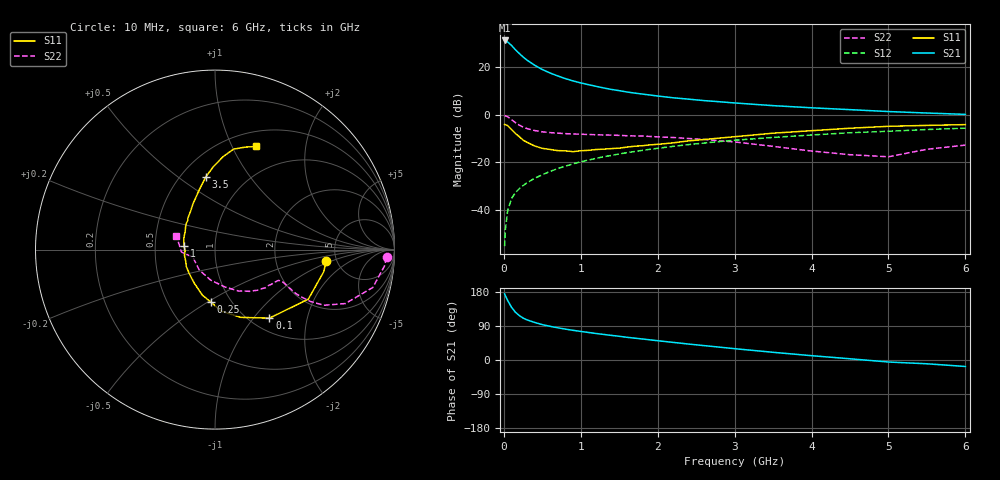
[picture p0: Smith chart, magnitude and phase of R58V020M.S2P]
! SIEMENS Small Signal Semiconductors
! BFR183
! Si NPN RF Bipolar Junction Transistor in SOT23
! VCE = 8 V  IC = 20 mA
! Common Emitter S-Parameters:  May  1996
# GHz  S  MA  R  50
!  f  S11  S21  S12  S22
! GHz  MAG  ANG  MAG  ANG  MAG  ANG  MAG  ANG
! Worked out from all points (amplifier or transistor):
!   36 points, 10 MHz to 6 GHz, reference 50 ohm
!   highest |S21| = 31.3 dB at 10 MHz (marker M1)
!   |S21| within 3 dB of that: start of sweep to 125 MHz
!   unconditionally stable (mu >= 1): 633.2 MHz to 2.498 GHz
!   at 250 MHz: K = 0.78, MSG = 27.1 dB, |S12| = -29.9 dB
!   at 1.4 GHz: K = 1.04, MAG = 12.6 dB, |S12| = -17.2 dB
!   at 6 GHz: K = 0.90, MSG = 2.9 dB, |S12| = -5.7 dB
!   S11 on the Smith chart (normalised r, x): 10 MHz: 4.12, -0.83; 100 MHz: 1.21, -1.21; 250 MHz: 0.81, -0.51; 1 GHz: 0.70, +0.03; 3.5 GHz: 0.66, +0.64; 6 GHz: 0.67, +1.24
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0.01  0.6227 -5.7  36.67 174.4  0.0017 78.0  0.9571 -2.6
0.02  0.6182 -11.5  36.16 169.7  0.0038 88.4  0.9483 -5.6
0.05  0.5886 -28.0  34.08 156.9  0.0096 79.0  0.9041 -13.5
0.1  0.4874 -51.6  28.73 139.1  0.0172 72.5  0.7856 -22.5
0.15  0.4038 -69.2  23.46 126.1  0.0228 68.1  0.681 -27.1
0.2  0.3457 -83.9  19.54 117.4  0.0276 67.5  0.6054 -28.5
0.25  0.2923 -94.8  16.47 110.7  0.0321 67.6  0.5486 -28.7
0.3  0.263 -105.6  14.16 105.9  0.0367 69.1  0.5112 -28.5
0.4  0.2197 -121.8  11.04 99.1  0.0457 69.9  0.4645 -27.2
0.5  0.1955 -137.6  8.96 93.3  0.0543 70.3  0.4364 -26.2
0.6  0.1856 -149.5  7.577 88.9  0.0639 70.9  0.4198 -25.6
0.7  0.1753 -158.7  6.562 85.0  0.0731 70.9  0.4087 -25.6
0.8  0.1732 -169.2  5.759 81.5  0.0825 70.3  0.3993 -25.7
1  0.1742 173.1  4.672 75.4  0.1017 69.5  0.3884 -26.7
1.1  0.1776 167.3  4.294 72.7  0.1111 68.9  0.3833 -27.8
1.3  0.1882 155.2  3.656 67.4  0.1304 67.2  0.374 -29.5
1.6  0.2078 142.0  3.013 59.9  0.1584 64.5  0.3604 -33.4
2.2  0.2551 122.0  2.275 46.5  0.2153 58.4  0.3314 -42.9
3.5  0.4082 97.2  1.552 20.3  0.332 42.3  0.2152 -75.2
4.5  0.5191 85.1  1.278 3.2  0.4166 30.0  0.1436 -127.8
5.5  0.5956 73.5  1.085 -10.0  0.4871 18.7  0.187 -175.7
6  0.6184 68.3  1.016 -17.1  0.5208 11.3  0.229 160.2
